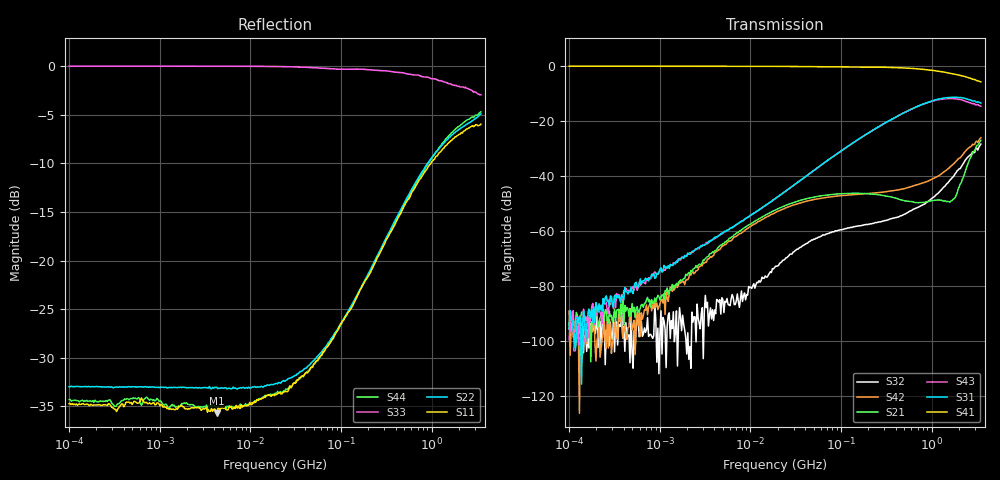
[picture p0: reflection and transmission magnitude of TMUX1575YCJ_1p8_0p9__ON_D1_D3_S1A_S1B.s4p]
!Keysight Technologies,E5080A,MY55200740,A.12.60.03
!Date: Wednesday, July 22, 2020 12:06:28
!Correction: S11(Full 4 Port(1,2,3,4))
!S12(Full 4 Port(1,2,3,4))
!S13(Full 4 Port(1,2,3,4))
!S14(Full 4 Port(1,2,3,4))
!S21(Full 4 Port(1,2,3,4))
!S22(Full 4 Port(1,2,3,4))
!S23(Full 4 Port(1,2,3,4))
!S24(Full 4 Port(1,2,3,4))
!S31(Full 4 Port(1,2,3,4))
!S32(Full 4 Port(1,2,3,4))
!S33(Full 4 Port(1,2,3,4))
!S34(Full 4 Port(1,2,3,4))
!S41(Full 4 Port(1,2,3,4))
!S42(Full 4 Port(1,2,3,4))
!S43(Full 4 Port(1,2,3,4))
!S44(Full 4 Port(1,2,3,4))
!S4P File: Measurements: <S11,S12,S13,S14>,
!<S21,S22,S23,S24>,
!<S31,S32,S33,S34>,
!<S41,S42,S43,S44>:Log Frequency Sweep
# Hz S  dB  R 50
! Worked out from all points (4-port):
!   400 points, 100 kHz to 3.5 GHz, reference 50 ohm
!   strongest paths, dB at 100 kHz, 1.377 MHz, 18.96 MHz, 261 MHz, 3.5 GHz:
!     S41: -0.2, -0.2, -0.2, -0.5, -5.9
!     S31: -95.4, -72.4, -48.2, -22.1, -13.6
!     S43: -99.4, -72.5, -48.2, -22.1, -14.7
!     S21: -94.1, -79.4, -52.4, -46.8, -27.0
!     S42: -89.1, -81.9, -53.3, -46.0, -26.1
!     S32: -95.5, -95.4, -72.8, -56.7, -28.4
!   lowest |S11| = -35.7 dB at 4.252 MHz (marker M1), VSWR 1.03, Z = 51.6 - j0.531 ohm
!   |S11| at or under -10 dB: start of sweep to 980.9 MHz
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100000  -34.72 7.4  -88.65 49.1  -103.16 18.2  -0.16 -0.0
        -94.15 -176.6  -32.97 1.9  -103.99 157.6  -91.59 -147.6
        -95.44 179.9  -95.49 41.0  0.00 -0.0  -94.49 7.1
        -0.16 -0.0  -89.07 128.4  -99.39 108.4  -34.29 7.3
1489464  -35.34 -11.0  -80.25 103.7  -71.55 89.5  -0.15 -0.1
         -80.05 144.1  -33.05 -4.2  -94.58 90.9  -79.63 152.5
         -71.91 96.2  -96.81 61.8  0.00 -0.1  -71.34 92.7
         -0.15 -0.1  -80.38 126.0  -71.42 89.7  -35.10 -8.7
4251829  -35.71 -18.3  -66.62 104.9  -62.20 94.2  -0.16 -0.3
         -66.76 122.2  -33.03 -12.0  -86.45 111.3  -67.82 126.8
         -62.16 93.2  -84.84 99.9  -0.00 -0.3  -61.84 93.1
         -0.16 -0.3  -67.44 112.6  -62.27 93.4  -35.05 -14.7
1.245977e7  -34.31 -45.9  -55.54 80.7  -52.30 98.3  -0.19 -0.8
            -55.48 85.6  -33.02 -30.6  -79.97 112.5  -56.48 86.3
            -52.32 98.6  -78.01 110.5  -0.01 -1.0  -52.29 98.5
            -0.19 -0.8  -56.49 81.0  -52.30 98.2  -34.21 -44.6
4.746034e7  -30.99 -82.1  -47.85 38.9  -38.58 100.8  -0.29 -2.0
            -47.84 40.2  -30.49 -72.6  -63.45 73.1  -48.77 32.8
            -38.59 100.7  -63.23 73.1  -0.14 -3.8  -38.61 101.3
            -0.29 -2.0  -48.77 31.7  -38.61 101.3  -30.92 -82.6
1.593708e9  -7.77 -133.0  -49.51 101.2  -11.50 15.6  -2.70 -31.9
            -49.50 101.5  -7.31 -128.0  -41.50 -88.3  -36.78 -115.1
            -11.51 15.7  -41.52 -88.3  -1.81 -75.6  -11.90 32.3
            -2.69 -31.9  -36.77 -115.1  -11.89 32.2  -7.03 -121.2
3.5e9  -5.96 -156.6  -26.99 146.7  -13.62 -14.8  -5.92 -50.1
       -27.02 146.9  -4.89 -140.8  -28.45 -179.1  -26.16 177.6
       -13.58 -15.1  -28.43 -179.4  -2.93 -110.3  -14.70 37.2
       -5.88 -50.3  -26.13 177.4  -14.70 37.3  -4.70 -143.1
